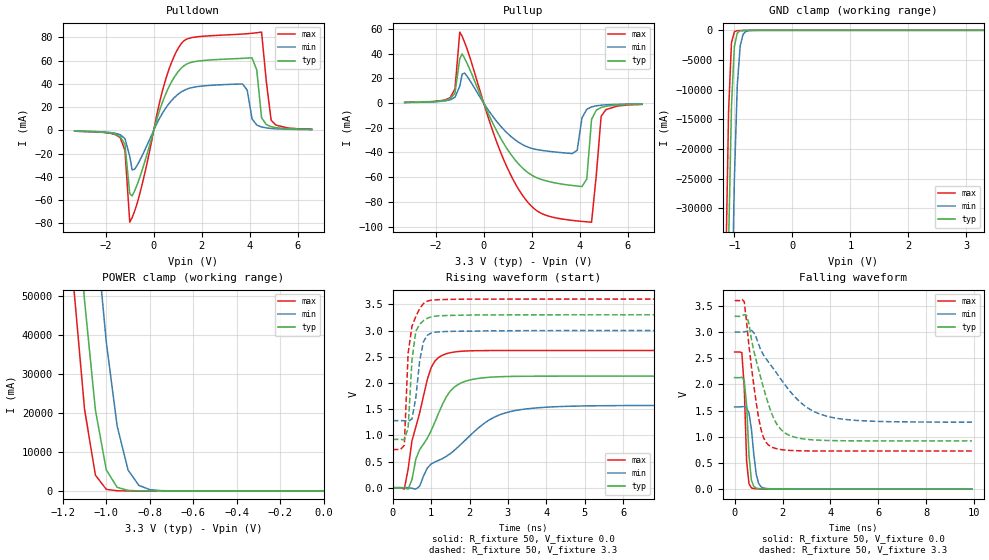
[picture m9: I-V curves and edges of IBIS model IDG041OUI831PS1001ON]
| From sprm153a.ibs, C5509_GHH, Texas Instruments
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| Pin_model   IDG041_OUI831_PS1001ON
[Model]   IDG041OUI831PS1001ON
 Model_type   I/O
 Polarity   Non-Inverting
 Enable   Active-Low
 Vinl  =  1.08
 Vinh  =  2.1
 Vmeas =  1.5
|Variable   typ   min   max
 C_comp   2.073pF   2.058pF   2.151pF
[Temperature Range]   25   125   -40
[Voltage Range]   3.3   3   3.6
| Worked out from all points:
|   slope of the pulldown table from 0 to 0.495 V, typ, clamps not added: 16 ohm
|   slope of the pullup table from 0 to 0.495 V, typ, clamps not added: 23.8 ohm
|   GND clamp passes 1 mA (typ) near -0.58 V on its own axis
|   POWER clamp passes 1 mA (typ) near -0.70 V on its own axis
|   rising waveform, R_fixture 50, V_fixture 0.0: 20-80 % time 803ps typ, 1.58ns min, 482ps max; typ from 0.001 V to 2.13 V
|   rising waveform, R_fixture 50, V_fixture 3.3: 20-80 % time 151ps typ, 187ps min, 161ps max; typ from 0.923 V to 3.3 V
|   falling waveform, R_fixture 50, V_fixture 0.0: 20-80 % time 167ps typ, 229ps min, 123ps max; typ from 2.13 V to 0.001 V
|   falling waveform, R_fixture 50, V_fixture 3.3: 20-80 % time 871ps typ, 1.74ns min, 493ps max; typ from 3.3 V to 0.923 V
[GND Clamp]
|Voltage   I(typ)   I(min)   I(max)
-3.3V     -2.131kA   -2.172kA   -2.112kA
-1.15V    -69.25A    -121A      -41.3A
-1.1V     -36.04A    -83.7A     -13.64A
-1.05V    -12.77A    -50.83A    -2.067A
-1V       -2.726A    -25.08A    -235.9mA
-950mV    -452.8mA   -9.272A    -58.97mA
-900mV    -87.55mA   -2.634A    -35.49mA
-850mV    -29.08mA   -661.8mA   -25.54mA
-800mV    -15.85mA   -165.5mA   -17.57mA
-600mV    -1.26mA    -2.585mA   -943.3uA
3.3V      224.3pA    17.39uA    -31.53uA
[POWER Clamp]
|Voltage   I(typ)   I(min)   I(max)
-3.3V     2.152kA    2.199kA    2.128kA
-1.15V    84.65A     142.8A     52.53A
-1.1V     48.8A      103.8A     20.98A
-1.05V    20.76A     68.2A      4.051A
-1V       5.397A     38.14A     409.1mA
-950mV    921.2mA    16.63A     39.38mA
-900mV    138.6mA    5.377A     6.941mA
-850mV    22.06mA    1.408A     3.332mA
-800mV    4.689mA    339.9mA    2.315mA
-750mV    1.723mA    80.98mA    1.625mA
0V        0A         0A         0A
[Pulldown]
|Voltage   I(typ)   I(min)   I(max)
-3.3V     -700uA     -600uA     -800uA
-1.4V     -5.36mA    -3.81mA    -6.27mA
-1.2V     -12.24mA   -7.1mA     -17.31mA
-1V       -54.58mA   -22.44mA   -78.99mA
-800mV    -52.16mA   -33.54mA   -69.68mA
400mV     26.07mA    15.89mA    36.64mA
1.1V      52.31mA    32.25mA    73.11mA
3.7V      61.86mA    39.87mA    82.75mA
4.1V      62.32mA    9.97mA     83.41mA
4.5V      10.72mA    2.83mA     84.43mA
4.9V      3.13mA     1.59mA     8.65mA
6.6V      700uA      600uA      1mA
[Pullup]
|Voltage   I(typ)   I(min)   I(max)
-3.3V     500uA      500uA      600uA
-1.4V     3.68mA     2.67mA     4.46mA
-1.2V     7.89mA     4.73mA     11.41mA
-1V       35.94mA    13.64mA    57.52mA
850mV     -33.18mA   -21.68mA   -46.54mA
2.15V     -59.85mA   -37.37mA   -86.19mA
3.7V      -66.75mA   -40.84mA   -95.02mA
4.1V      -67.58mA   -12.01mA   -95.82mA
4.3V      -61.52mA   -5.05mA    -96.15mA
4.5V      -13.11mA   -3.07mA    -96.45mA
4.9V      -3.53mA    -1.69mA    -10.6mA
6.6V      -800uA     -600uA     -1.1mA
[Ramp]
|Variable   typ   min   max
 dV/dt_r   1.29V/0.810ns   0.95V/1.590ns   1.59V/0.490ns
 dV/dt_f   1.44V/0.880ns   1.04V/1.750ns   1.72V/0.490ns
 R_load =  50
[Rising Waveform]
 R_fixture =   50
 V_fixture =   0.0
 V_fixture_min =  0.0
 V_fixture_max =  0.0
|Time   V(typ)   V(min)   V(max)
0s        1.035mV    903.9uV    1.259mV
300ps     503.6uV    2.198mV    -25.47mV
500ps     151.8mV    -10.49mV   897.6mV
600ps     545.4mV    -26.24mV   1.158V
900ps     945.6mV    376mV      2.066V
1.1ns     1.258V     493.6mV    2.419V
1.4ns     1.741V     601mV      2.559V
2ns       2.054V     986.9mV    2.612V
3.3ns     2.126V     1.486V     2.619V
9.9ns     2.129V     1.57V      2.619V
[Rising Waveform]
 R_fixture =   50
 V_fixture =   3.3
 V_fixture_min =  3
 V_fixture_max =  3.6
|Time   V(typ)   V(min)   V(max)
0s        922.7mV    1.28V      729.2mV
300ps     912.9mV    1.28V      808.1mV
400ps     1.143V     1.264V     2.568V
500ps     2.434V     1.313V     3.081V
600ps     2.985V     1.715V     3.265V
700ps     3.119V     2.415V     3.418V
800ps     3.189V     2.788V     3.514V
900ps     3.233V     2.91V      3.561V
1.8ns     3.292V     2.987V     3.597V
9.9ns     3.3V       3V         3.6V
[Falling Waveform]
 R_fixture =   50
 V_fixture =   0.0
 V_fixture_min =  0.0
 V_fixture_max =  0.0
|Time   V(typ)   V(min)   V(max)
0s        2.129V     1.57V      2.619V
300ps     2.136V     1.574V     2.608V
400ps     2.08V      1.578V     1.956V
500ps     1.597V     1.552V     529.9mV
600ps     633.1mV    1.451V     103.8mV
700ps     171.2mV    1.146V     24.82mV
900ps     22.38mV    287.5mV    9.227mV
1ns       13.02mV    111.5mV    7.571mV
1.2ns     7.93mV     23.39mV    5.507mV
9.9ns     1.034mV    903.4uV    1.259mV
[Falling Waveform]
 R_fixture =   50
 V_fixture =   3.3
 V_fixture_min =  3
 V_fixture_max =  3.6
|Time   V(typ)   V(min)   V(max)
0s        3.3V       3V         3.6V
400ps     3.331V     3.003V     3.58V
600ps     3.15V      3.027V     2.726V
1ns       2.284V     2.768V     1.364V
1.2ns     1.944V     2.565V     990.4mV
1.5ns     1.5V       2.374V     816.6mV
2.2ns     1.046V     1.933V     743.5mV
3ns       953.2mV    1.567V     731.1mV
3.8ns     931mV      1.399V     729.2mV
9.9ns     922.7mV    1.28V      729.2mV
